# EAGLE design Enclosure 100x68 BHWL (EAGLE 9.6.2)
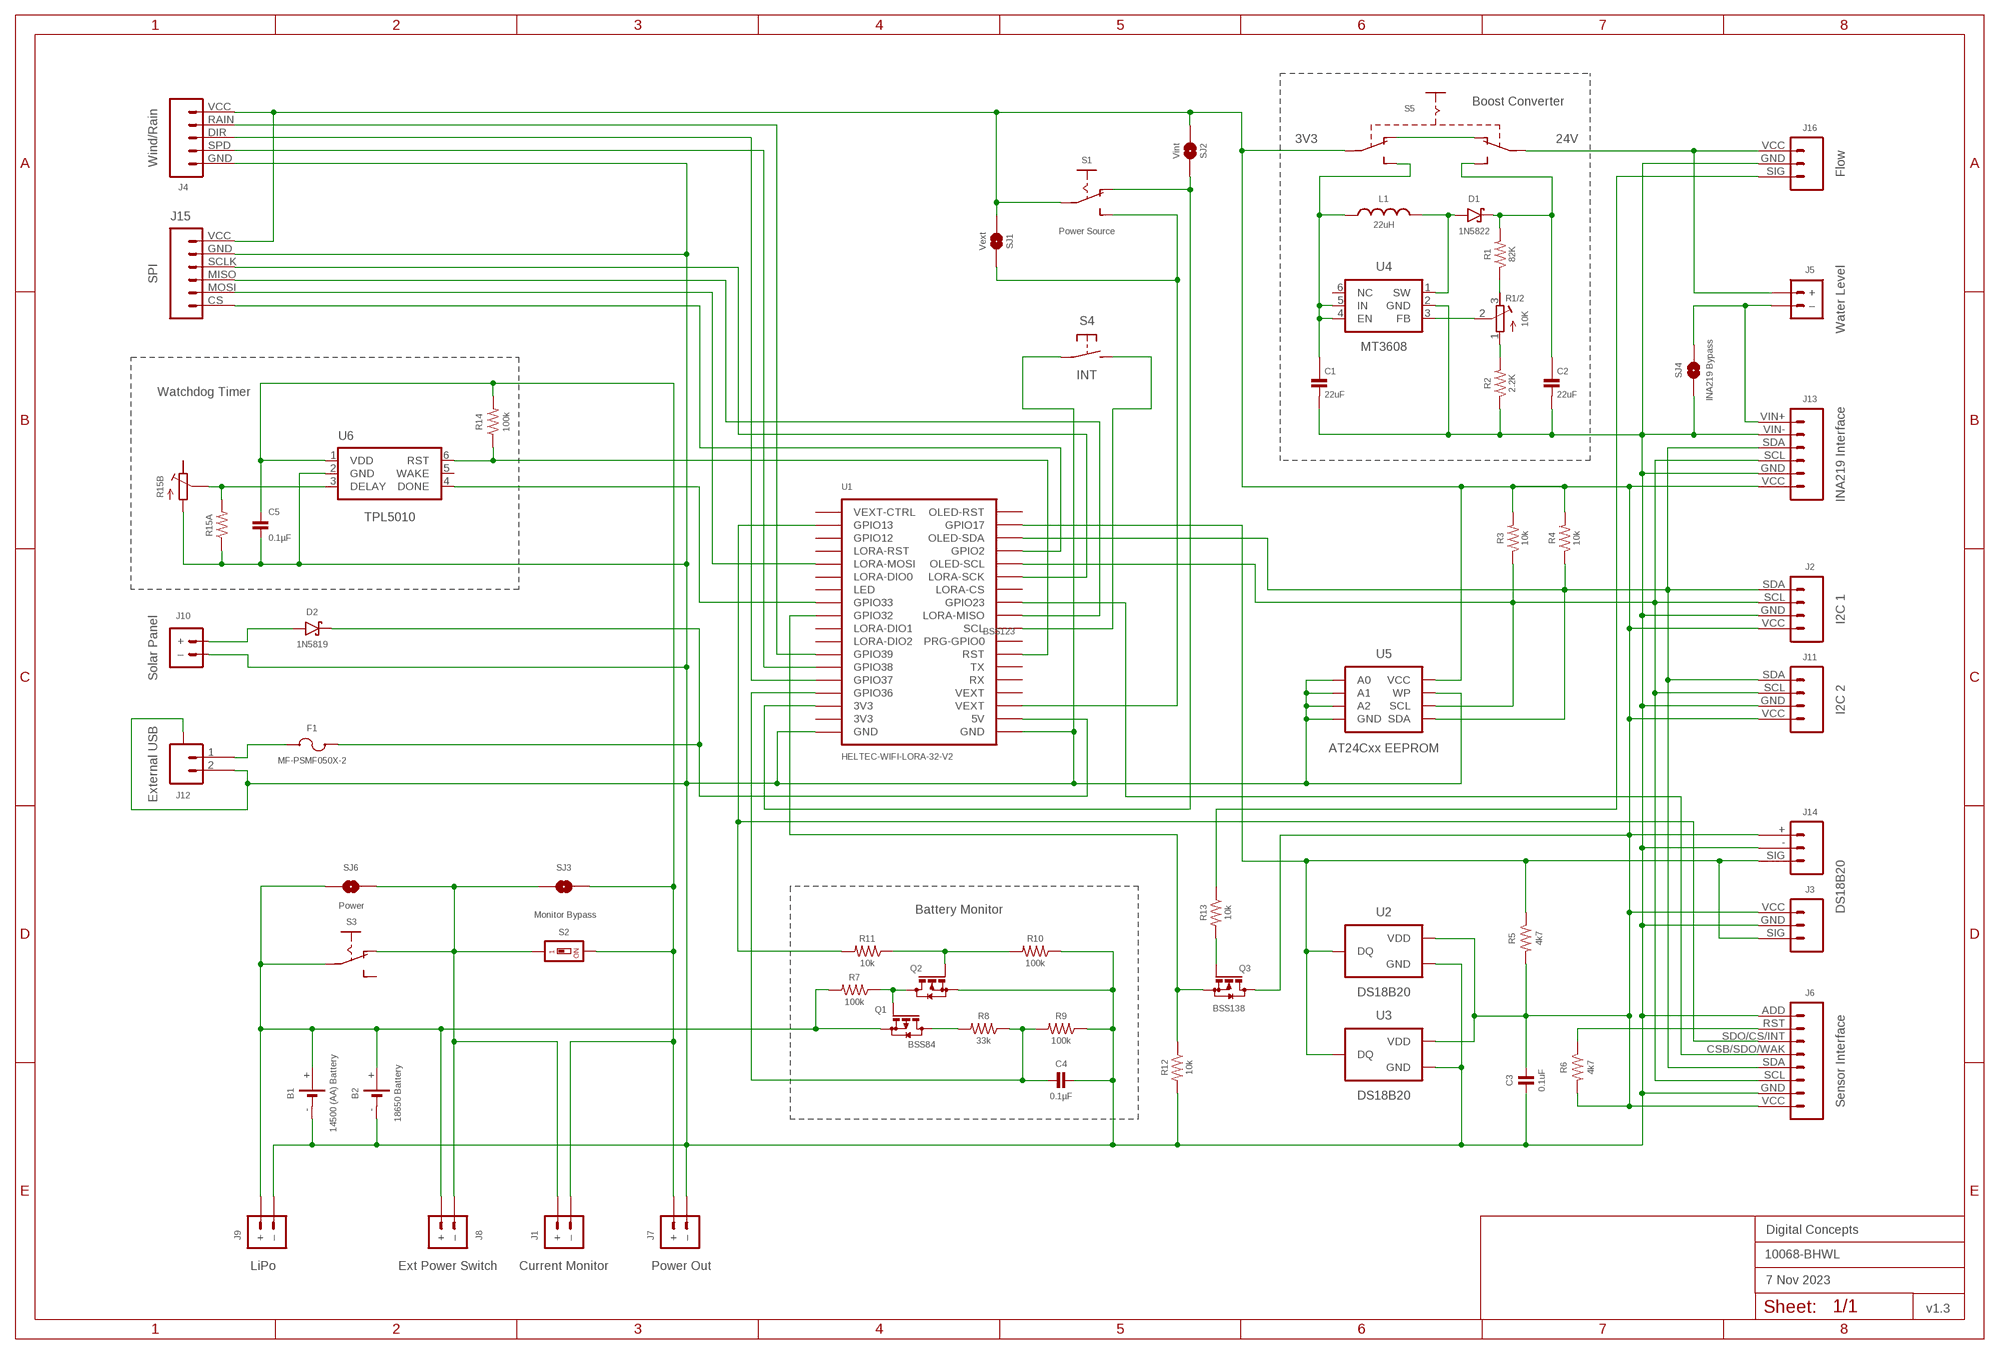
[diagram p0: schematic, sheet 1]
FRAME2 (A3L-LOC): DATE: 7 Nov 2023; OWNER: Digital Concepts; TITLE: 10068-BHWL; VERSION: v1.3

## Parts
B1  14500 (AA) Battery  BATTERY-HOLDER-14500(AA)  [BATTERY-14500]
B2  18650 Battery  BATTERY-HOLDER-18650  [BATTERY-18650]
C1  22uF  CAPACITOR-1206  [C1206]
C2  22uF  CAPACITOR-1206  [C1206]
C3  0.1uF  CAPACITOR-0805  [C0805]
C4  0.1µF  CAPACITOR-0805  [C0805]
C5  0.1µF  CAPACITOR-0805  [C0805]
D1  1N5822  DIODE-SCHOTTKY-1N5822  [DIODE_SMB]
D2  1N5819  1N5819-SOD-123  [SOD-123]
F1  MF-PSMF050X-2  [F0805]
J1  Current Monitor  JST-PH2.0-2-HORIZONTALJST-PTH-2  [JST-PH2.0-2-HORIZONTAL]
J2  I2C 1  JST-PH2.0-4-VERTICAL-I2C  [JST-PH2.0-4-VERTICAL-I2C]
J3  DS18B20  JST-PH2.0-3-VERTICAL-DS18B20  [JST-PH2.0-3-VERTICAL-SIG]
J4  Wind/Rain  JST-PH2.0-5-DUAL-WEATHER  [JST-PH2.0-5-DUAL-WEATHER]
J5  Water Level  JST-PH2.0-2-DUAL-POWERJST-PTH-2  [JST-PH2.0-2-DUAL-POWER]
J6  Sensor Interface  HEADER-1X8-SENSOR  [CONN_08-SENSOR]
J7  Power Out  JST-GH1.25-2-HORIZONTAL-POWER  [JST-GH1.25-2-HORIZONTAL]
J8  Ext Power Switch  JST-PH2.0-2-DUAL-POWERJST-PTH-2  [JST-PH2.0-2-DUAL-POWER]
J9  LiPo  JST-PH2.0-2-HORIZONTAL-POWERJST-PTH-2  [JST-PH2.0-2-HORIZONTAL-POWER]
J10  Solar Panel  JST-PH2.0-2-VERTICAL  [JST-PH2.0-2-VERTICAL=POWER]
J11  I2C 2  JST-PH2.0-I2C-MALE-HORIZONTAL  [JST-PH2.0-4-HORIZONTAL]
J12  External USB  JST-SH1.0-2-SMD-HORIZONTAL  [JST-SH1.0-2-HORIZONTAL]
J13  INA219 Interface  INA219-I2C-MODULE  [CONN_06-INA219]
J14  JST-PH2.0-3-HORIZONTAL-DS18B20  [JST-PH2.0-3-HORIZONTAL-DS18B20]
J15  SPI  JST-PH2.0-6-HORIZONTAL-SPI  [JST-PH2.0-6-HORIZONTAL-SPI]
J16  Flow  JST-XH2.54-3-VERTICAL-SENSOR  [JST-XH2.4-3-VERTICAL-SENSOR]
L1  22uH  INDUCTOR-CDRH104R/6D28L5038P  [CDRH104R+6D28]
Q1  BSS84  [SOT23-3]
Q2  BSS123  MOSFET-BSS123  [SOT23-3]
Q3  BSS138  MOSFET-BSS123  [SOT23-3]
R1  82K  RESISTORR0805  [R0805]
R1/2  10K  RESISTOR-TRIMM-BAOTER-HORIZONTAL  [RTRIM64P]
R2  2.2K  RESISTORR0805  [R0805]
R3  10k  RESISTORR0805  [R0805]
R4  10k  RESISTORR0805  [R0805]
R5  4k7  RESISTORR0805  [R0805]
R6  4k7  RESISTORR0805  [R0805]
R7  100k  RESISTORR0805  [R0805]
R8  33k  RESISTORR0805  [R0805]
R9  100k  RESISTORR0805  [R0805]
R10  100k  RESISTORR0805  [R0805]
R11  10k  RESISTORR0805  [R0805]
R12  10k  RESISTORR0805  [R0805]
R13  10k  RESISTORR0805  [R0805]
R14  100k  RESISTORR0805  [R0805]
R15A  RESISTORR0805  [R0805]
R15B  RESISTOR-TRIMM-33  [RTRIM3*3]
S1  Power Source  SWITCH-SLIDE-SPDT-SMT  [SWITCH-SPDT-SMT]
S2  Monitor Bypass  SWITCH-DIP-SWS001  [SMD-001]
S3  Power  SWITCH-SLIDE-SPDT-PTH  [SWITCH-SPDT-PTH]
S4  INT  SWITCH-MOMENTARY-2-PIN  [SWITCH-2-PAD]
S5  SWITCH-SLIDE-DPDT-PTH-S  [SWITCH-DPDT-PTH]
SJ1  Vext  SJ  [SJ]
SJ2  Vint  SJ-V-2  [SJ-VIA-2]
SJ3  Monitor  SJ  [SJ]
SJ4  INA219 Bypass  SJ  [SJ]
SJ6  Power  SJ  [SJ]
U1  HELTEC-WIFI-LORA-32-V2  [HELTEC-WIFI-LORA-32-V2]
U2  DS18B20  THERMOMETER-DS18B20  [TO-92]
U3  DS18B20  THERMOMETER-DS18B20  [TO-92]
U4  MT3608  [SOT-23-6@1]
U5  AT24Cxx EEPROM  AT24CXX-EEPROM  [SOP-8]
U6  TPL5010  TPL5010DDCR  [SOT-23-6]

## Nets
GND: B1.- B2.- C1.2 C2.2 C3.2 C4.2 C5.2 J2.GND J3.GND J4.GND J6.ADD J6.GND J7.-(–) J9.-(–) J10.-(–) J11.GND J12.2 J12.A@1(A) J12.A@2(A) J13.GND J13.VIN- J14.- J15.GND J16.GND Q2.2(S) R2.1 R9.1 R10.1 R12.2 R15A.1 R15B.1(A) S4.P$1(P) SJ4.1 U1.GND@1(GND) U1.GND@36(GND) U2.1(GND) U3.1(GND) U4.2(GND) U5.P$1(A0) U5.P$2(A1) U5.P$3(A2) U5.P$4(GND) U5.P$7(WP) U6.2(GND)
N$1: D2.A J10.+
N$2: J4.RAIN U1.GPIO39
N$3: J6.CSB/SDO/WAK U1.GPIO23
N$4: J2.SCL J6.SCL J11.SCL J13.SCL R3.1 U1.GPIO15(OLED-SCL) U5.P$6(SCL)
N$5: D2.C F1.1 U1.5V
N$6: D1.A L1.1 U4.1(SW)
N$7: Q1.3(D) R8.2
N$8: C5.1 J1.2(–) J7.+ R14.2 S2.2 SJ3.1 U6.1(VDD)
N$9: J6.RST R6.1
N$10: J4.DIR U1.GPIO37
N$11: J2.SDA J6.SDA J11.SDA J13.SDA R4.1 U1.GPIO4(OLED-SDA) U5.P$5(SDA)
N$12: J4.SPD U1.GPIO38
N$13: S1.3(S) SJ1.1 U1.VEXT@3(VEXT)
N$14: F1.2 J12.1
N$15: J5.-(–) J13.VIN+ SJ4.2
N$16: R1.1 R1/2.3(E)
N$17: S4.P$2(S) U1.GPIO22(SCL)
N$18: C4.1 R8.1 R9.2 U1.GPIO36
N$19: S1.1(O) SJ2.1 U1.3V3@34(3V3)
N$20: J5.+ J16.VCC S5.P$2(P1)
N$21: J1.1(+) J8.-(–) S2.1 S3.1(O) SJ3.2 SJ6.1
N$22: R1/2.2(S) U4.3(FB)
N$23: R1/2.1(A) R2.2
N$24: J3.SIG J14.SIG R5.1 U1.GPIO17 U2.2(DQ) U3.2(DQ)
N$25: C1.1 L1.2 S5.P$6(S2) U4.4(EN) U4.5(IN)
N$26: S5.P$1(O1) S5.P$4(O2)
N$27: J15.SCLK U1.GPIO5(LORA-SCK)
N$28: C2.1 D1.C R1.2 S5.P$3(S1)
N$29: J15.MOSI U1.GPIO27(LORA-MOSI)
N$30: B1.+ B2.+ J8.+ J9.+ Q1.2(S) R7.2 S3.2(P) SJ6.2
N$31: J15.MISO U1.GPIO19(LORA-MISO)
N$32: J6.SDO/CS/INT R11.2 U1.GPIO13
N$33: J15.CS U1.GPIO2
N$34: Q3.1(G) R13.2
N$35: Q1.1(G) Q2.3(D) R7.1
N$36: R15A.2 R15B.2(S) U6.3(DELAY)
N$37: Q2.1(G) R10.2 R11.1
N$38: R14.1 U1.RST U6.6(RST)
N$39: U1.GPIO33 U6.4(DONE)
N$40: Q3.2(S) R12.1 U1.GPIO32
N$42: J16.SIG R13.1
VEXT: C3.1 J2.VCC J3.VCC J4.VCC J6.VCC J11.VCC J13.VCC J14.+ J15.VCC Q3.3(D) R3.2 R4.2 R5.2 R6.2 S1.2(P) S5.P$5(P2) SJ1.2 SJ2.2 SJ2.2@V U2.3(VDD) U3.3(VDD) U5.P$8(VCC)
Unconnected: R15B.3(E) S3.3(S) U1.3V3@35(3V3) U1.GPIO0(PRG-GPIO0) U1.GPIO12 U1.GPIO14(LORA-RST) U1.GPIO16(OLED-RST) U1.GPIO18(LORA-CS) U1.GPIO21(VEXT-CTRL) U1.GPIO25(LED) U1.GPIO26(LORA-DIO0) U1.GPIO34(LORA-DIO2) U1.GPIO35(LORA-DIO1) U1.RX U1.TX U1.VEXT@4(VEXT) U4.6(NC) U6.5(WAKE)

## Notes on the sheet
- Boost Converter
- 3V3 | 24V
- Watchdog Timer
- Battery Monitor

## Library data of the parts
B1 = digitalconcepts:BATTERY-HOLDER-14500(AA): 14500 (AA) battery holder
B2 = digitalconcepts:BATTERY-HOLDER-18650: 18650 Battery Holder
C1 C2 = digitalconcepts:CAPACITOR-1206: 1206 Capacitor
C3-C5 = digitalconcepts:CAPACITOR-0805: 0805 Capacitor
D1 = digitalconcepts:DIODE-SCHOTTKY-1N5822: 1N5822 Schottky Diode SMB
D2 = digitalconcepts:1N5819-SOD-123: 1N5819 Schottky Diode SOD-123
F1 = digitalconcepts:MF-PSMF050X-2: PTC Resettable Fuse
J1 = digitalconcepts:JST-PH2.0-2-HORIZONTAL: PH2.0 2P Right Angle PCB Connector; PROD_ID: CONN-09863; SKU: PRT-09914
J2 = digitalconcepts:JST-PH2.0-4-VERTICAL-I2C: PH2.0 4P I2C Vertical Connector
J3 = digitalconcepts:JST-PH2.0-3-VERTICAL-DS18B20: DS18B20 PH2.0 Vertical PCB Connector
J4 = digitalconcepts:JST-PH2.0-5-DUAL-WEATHER: PH2.0 5P Dual Connector
J5 J8 = digitalconcepts:JST-PH2.0-2-DUAL-POWER: JST PH2.0 2P PTH Dual-Side Connector (Power); PROD_ID: CONN-09863; SKU: PRT-09914
J6 = digitalconcepts:HEADER-1X8-SENSOR: IoT Sensors 1x8 Pin Header for 'Sandwich' IoT Sensors
J7 = digitalconcepts:JST-GH1.25-2-HORIZONTAL-POWER: JST GH1.25 2P PTH Connector (Power)
J9 = digitalconcepts:JST-PH2.0-2-HORIZONTAL-POWER: PH2.0 2P Right Angle PCB Connector; PROD_ID: CONN-09863; SKU: PRT-09914
J10 = digitalconcepts:JST-PH2.0-2-VERTICAL: PH2.0 2P PCB Connector
J11 = digitalconcepts:JST-PH2.0-I2C-MALE-HORIZONTAL: PH2.0 4P (I2C) Right Angle PCB Connector
J12 = digitalconcepts:JST-SH1.0-2-SMD-HORIZONTAL: JST SH1.0 2P SMD Horizontal Connector
J13 = digitalconcepts:INA219-I2C-MODULE: INA219 I2C Module
J14 = digitalconcepts:JST-PH2.0-3-HORIZONTAL-DS18B20: DS18B20 PH2.0 Right Angle PCB Connector
J15 = digitalconcepts:JST-PH2.0-6-HORIZONTAL-SPI: PH2.0 6P Horizontal Connector—SPI
J16 = digitalconcepts:JST-XH2.54-3-VERTICAL-SENSOR: XH2.54 3P Vertical Connector with Sensor Labels
L1 = digitalconcepts:INDUCTOR-CDRH104R/6D28: Inductor; SPICEPREFIX: L
Q1 = digitalconcepts:BSS84: P-CHANNEL MOS FET
Q2 Q3 = digitalconcepts:MOSFET-BSS123: N-CHANNEL MOS FET
R1-R14 R15A = digitalconcepts:RESISTOR: Resistor; SPICEPREFIX: R
R1/2 = digitalconcepts:RESISTOR-TRIMM-BAOTER-HORIZONTAL: Trimm Resistor - Horizontal BAOTER
R15B = digitalconcepts:RESISTOR-TRIMM-3*3: Trimm Resistor - 3*3 SMD
S1 = digitalconcepts:SWITCH-SLIDE-SPDT-SMT: Mini Sliding Switch SPDT SMT
S2 = digitalconcepts:SWITCH-DIP-SWS001: SMD Dip Switch 1 pol.
S3 = digitalconcepts:SWITCH-SLIDE-SPDT-PTH: Mini Sliding Switch SPDT PTH
S4 = digitalconcepts:SWITCH-MOMENTARY-2-PIN: 2 Pin Momentary Switch
S5 = digitalconcepts:SWITCH-SLIDE-DPDT-PTH-S: Switch DPDT PTH-S
SJ1 SJ3 SJ4 SJ6 = digitalconcepts:SJ: Solder Jumper
SJ2 = digitalconcepts:SJ-V-2: Solder Jumper with Pad Vias
U1 = digitalconcepts:HELTEC-WIFI-LORA-32-V2: Heltec WiFi LoRa 32 Development Board V2
U2 U3 = digitalconcepts:THERMOMETER-DS18B20: Digital Thermometer -55C-125C TO92-3; AVAILABILITY: Bad; DESCRIPTION: Temperature Sensor Digital, Local -55°C ~ 125°C 12 b 8-uMAX; MF: Maxim Integrated; MP: DS18B20; PACKAGE: TO-92 Maxim Integrated; PRICE: None
U4 = digitalconcepts:MT3608: MT3608 DC-DC Step-Up Voltage Converter
U5 = digitalconcepts:AT24CXX-EEPROM: AT24Cxx EEPROM SOP-8
U6 = digitalconcepts:TPL5010DDCR: TPL5010 Nano-Power System Timer with Watchdog

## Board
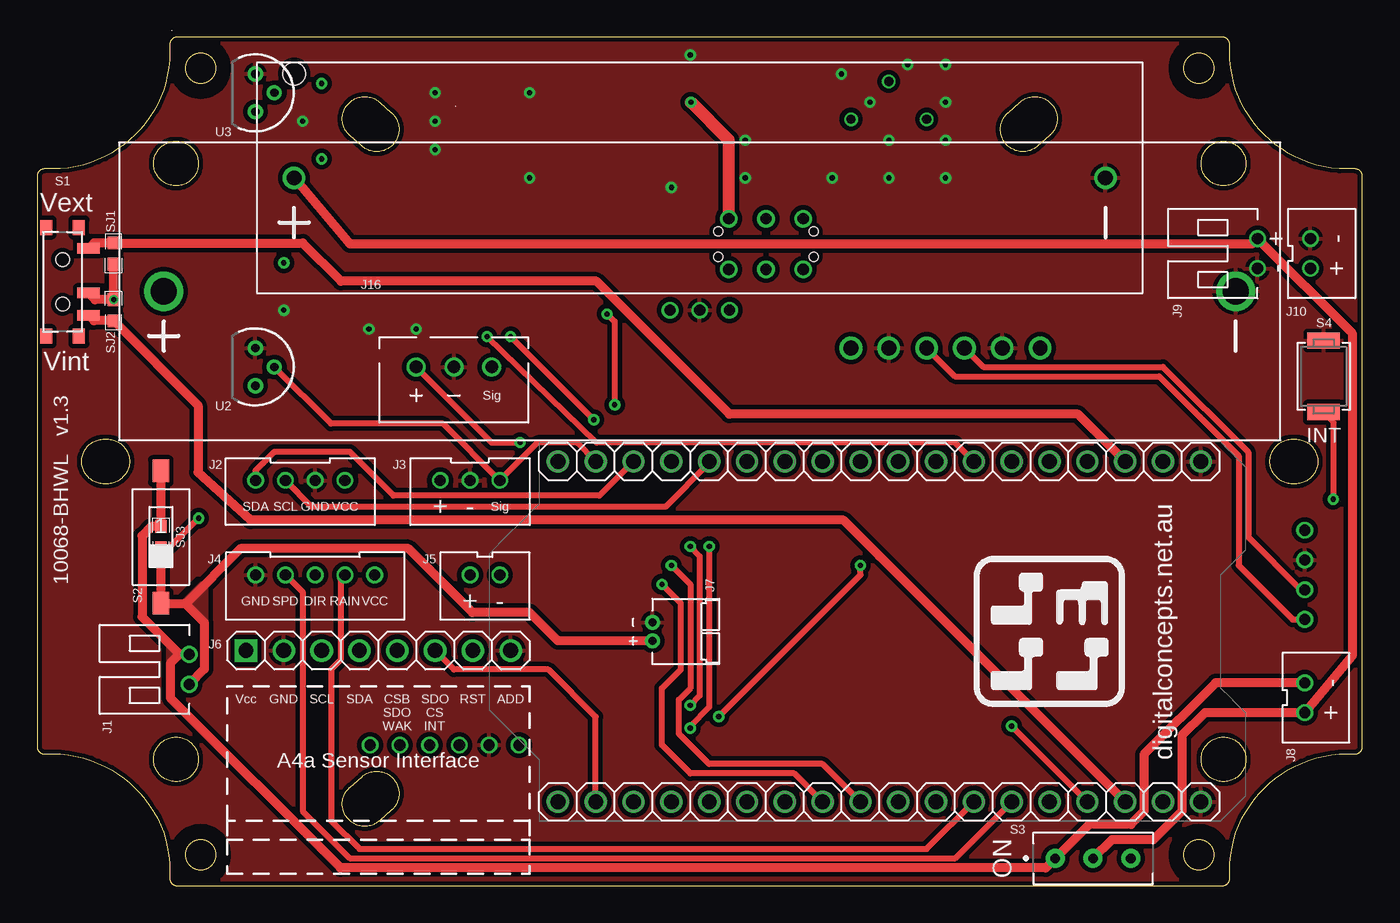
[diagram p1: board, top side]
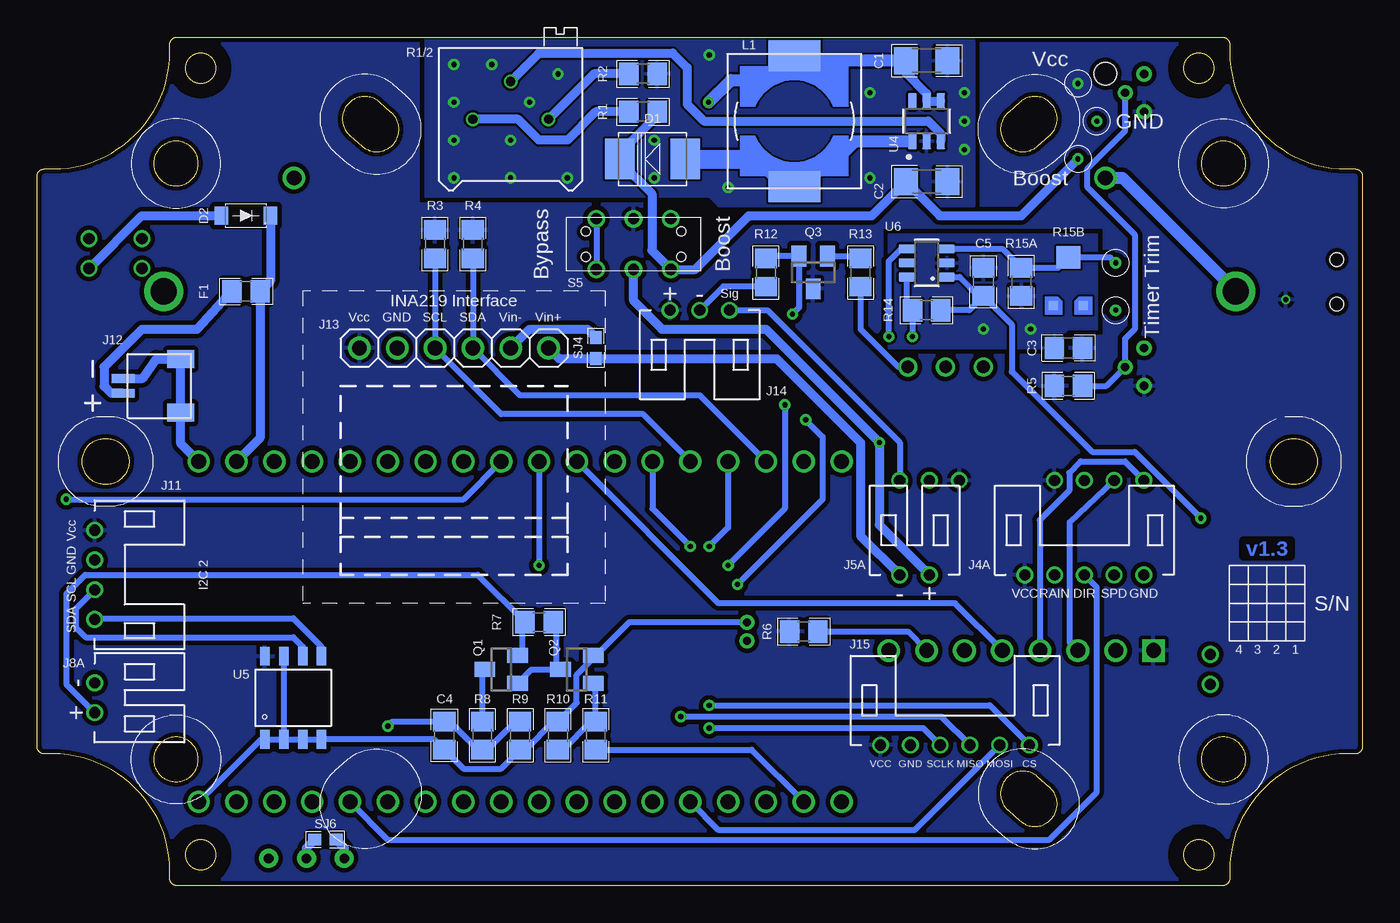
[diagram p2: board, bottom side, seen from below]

Size 89 x 57 mm. Coordinates in mm from the lower left corner, seen from the top.
Outline: 1134 segments
Outline: circle at 10.97,2.08 radius 1.02
Outline: circle at 10.97,54.92 radius 1.02
Outline: circle at 78.03,54.92 radius 1.02
Outline: circle at 78.03,2.08 radius 1.02
Copper layers (1*16): Top 0.035mm / dielectric 1.5mm / Bottom 0.035mm
Design rules "default *": minimum track width 6mil, minimum drill 0.35mm, track to track 6mil, track to pad 6mil, pad to pad 6mil, via to via 6mil, smd to smd 6mil, copper to edge 6mil, drill to drill 6mil, minimum pad ring 1mil, minimum via ring 8mil, stop-mask expansion 4mil, vias tented up to drill 0mil, thermal gap 10mil

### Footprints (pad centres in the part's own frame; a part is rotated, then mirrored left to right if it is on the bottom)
BATTERY-14500 = drill 1: + -27.25,0; - 27.25,0 | hole 1.524: -27.25,7
BATTERY-18650 = drill 1.75: + -36,0; - 36,0
C1206 = smd 1.6 x 1.8: 1 -1.4,0; 2 1.4,0
C0805 = smd 1.3 x 1.5: 1 -0.95,0; 2 0.95,0
DIODE_SMB = smd 2 x 2.7: A 2.2,0; C -2.2,0
SOD-123 = smd 0.91 x 1.22: A -1.65,0; C 1.65,0
F0805 = smd 1.3 x 1.5: 1 -0.95,0; 2 0.95,0
JST-PH2.0-2-HORIZONTAL = drill 0.75: 1 1,0; 2 -1,0
JST-PH2.0-4-VERTICAL-I2C = drill 0.75: GND 1,0; SCL -1,0; SDA -3,0; VCC 3,0
JST-PH2.0-3-VERTICAL-SIG = drill 0.75: GND 0,0; SIG 2,0; VCC -2,0
JST-PH2.0-5-DUAL-WEATHER = drill 0.75: DIR 0,0; GND 4,0; RAIN -2,0; SPD 2,0; VCC -4,0
JST-PH2.0-2-DUAL-POWER = drill 0.75: + 1,0; - -1,0
CONN_08-SENSOR = drill 1 pad 1.524: ADD 17.78,0; CSB/SDO/WAK 10.16,0; GND 2.54,0; RST 15.24,0; SCL 5.08,0; SDA 7.62,0; SDO/CS/INT 12.7,0 | drill 1 pad 1.524 square: VCC 0,0
JST-GH1.25-2-HORIZONTAL = drill 0.55 pad 1.016: + -0.625,0; - 0.625,0
JST-PH2.0-2-HORIZONTAL-POWER = drill 0.75: + 1,0; - -1,0
JST-PH2.0-2-VERTICAL=POWER = drill 0.75: + -1,0; - 1,0
JST-PH2.0-4-HORIZONTAL = drill 0.75: GND -1,0; SCL 1,0; SDA 3,0; VCC -3,0
JST-SH1.0-2-HORIZONTAL = smd 0.6 x 1.55: 1 -0.5,2.54; 2 0.5,2.54 | smd 1.2 x 1.8: A@1 -1.8,-1.335; A@2 1.8,-1.335
CONN_06-INA219 = drill 1 pad 1.524: GND 2.54,0; SCL 5.08,0; SDA 7.62,0; VCC 0,0; VIN+ 12.7,0; VIN- 10.16,0
JST-PH2.0-3-HORIZONTAL-DS18B20 = drill 0.75: + 2,0; - 0,0; SIG -2,0
JST-PH2.0-6-HORIZONTAL-SPI = drill 0.75: CS 5,0; GND -3,0; MISO 1,0; MOSI 3,0; SCLK -1,0; VCC -5,0
JST-XH2.4-3-VERTICAL-SENSOR = drill 0.85: GND 0,0; SIG 2.54,0; VCC -2.54,0
CDRH104R+6D28 = smd 2.1 x 3.5: 1 -4.4,0; 2 4.4,0
SOT23-3 = smd 1 x 1.4: 1 -0.95,-1.1; 2 0.95,-1.1; 3 0,1.1
R0805 = smd 1.3 x 1.5: 1 -0.95,0; 2 0.95,0
RTRIM64P = drill 0.61: 1 0,-2.54; 2 2.54,0; 3 0,2.54
RTRIM3*3 = smd 0.6 x 0.6: 1 -1,-1.6; 3 1,-1.6 | smd 1.6 x 1.5: 2 0,1.65
SWITCH-SPDT-SMT = smd 0.7 x 1.5: 1 2.25,1.75; 2 0.75,1.75; 3 -2.25,1.75 | smd 1 x 0.8: GND@1 3.65,-1.1; GND@2 3.65,1.1; GND@3 -3.65,1.1; GND@4 -3.65,-1.1 | hole 0.9: -1.5,0; 1.5,0
SMD-001 = smd 1.1 x 1.5: 1 0,-4.45; 2 0,4.45
SWITCH-SPDT-PTH = drill 0.65 pad 1.27: 1 -2.54,0; 2 0,0; 3 2.54,0
SWITCH-2-PAD = smd 1.067 x 2.184: P$1 -2.4,0; P$2 2.4,0
SWITCH-DPDT-PTH = drill 0.75 pad 1.19: P$1 -1.7,2.5; P$2 -1.7,0; P$3 -1.7,-2.5; P$4 1.7,2.5; P$5 1.7,0; P$6 1.7,-2.5 | hole 0.6: 0.85,3.2; -0.85,3.2; 0.85,-3.2; -0.85,-3.2
SJ = smd 0.864 x 0.762: 1 -0.711,0; 2 0.711,0
SJ-VIA-2 = smd 0.864 x 0.762: 1 -0.711,0; 2 0.711,0 | drill 0.35 pad 0.61: 2@V 0.711,0
HELTEC-WIFI-LORA-32-V2 = drill 1: 3V3@34 -22.86,5.08; 3V3@35 -22.86,2.54; 5V 0,2.54; GND@1 0,0; GND@36 -22.86,0; GPIO0 0,17.78; GPIO2 0,35.56; GPIO4 0,38.1; GPIO5 0,30.48; GPIO12 -22.86,38.1; GPIO13 -22.86,40.64; GPIO14 -22.86,35.56; GPIO15 0,33.02; GPIO16 0,43.18; GPIO17 0,40.64; GPIO18 0,27.94; GPIO19 0,22.86; GPIO21 -22.86,43.18; GPIO22 0,20.32; GPIO23 0,25.4; GPIO25 -22.86,27.94; GPIO26 -22.86,30.48; GPIO27 -22.86,33.02; GPIO32 -22.86,22.86; GPIO33 -22.86,25.4; GPIO34 -22.86,17.78; GPIO35 -22.86,20.32; GPIO36 -22.86,7.62; GPIO37 -22.86,10.16; GPIO38 -22.86,12.7; GPIO39 -22.86,15.24; RST 0,15.24; RX 0,10.16; TX 0,12.7; VEXT@3 0,5.08; VEXT@4 0,7.62
TO-92 = drill 0.55 pad 1.016: 1 -1.27,0; 2 0,1.27; 3 1.27,0
SOT-23-6@1 = smd 1.1 x 0.6: 1 -1.35,0.95; 2 -1.35,0; 3 -1.35,-0.95; 4 1.35,-0.95; 5 1.35,0; 6 1.35,0.95
SOP-8 = smd 0.635 x 1.27: P$1 -1.905,-2.794; P$2 -0.635,-2.794; P$3 0.635,-2.794; P$4 1.905,-2.794; P$5 1.905,2.794; P$6 0.635,2.794; P$7 -0.635,2.794; P$8 -1.905,2.794
SOT-23-6 = smd 1.1 x 0.6: 1 -1.35,0.95; 2 -1.35,0; 3 -1.35,-0.95; 4 1.35,-0.95; 5 1.35,0; 6 1.35,0.95

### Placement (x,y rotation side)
B1  44.5,47.55 0 top
B2  44.5,39.93 0 top
C1  29.26,55.42 0 bottom
C2  29.26,47.3 0 bottom
C3  19.73,36.12 180 bottom
C4  61.64,10.08 270 bottom
C5  25.45,40.56 90 bottom
D1  47.67,48.82 0 bottom
D2  74.98,45.01 0 bottom
F1  74.98,39.93 180 bottom
J1  10.21,14.53 90 top
J2  17.67,27.23 0 top
J3  29.07,27.23 0 top
J4  18.67,20.88 0 bottom
J5  30.07,20.88 0 bottom
J6  14.02,15.8 0 top
J7  41.32,17.07 90 top
J8  85.14,12.62 270 bottom
J9  81.96,42.47 90 top
J10  85.52,42.47 90 top
J11  85.14,20.88 270 bottom
J12  80.69,33.58 90 bottom
J13  67.36,36.12 0 bottom
J14  44.5,38.66 180 bottom
J15  27.35,9.45 0 bottom
J16  27.99,34.85 0 top
L1  38.15,51.36 90 bottom
Q1  57.83,14.53 90 bottom
Q2  52.75,14.53 90 bottom
Q3  36.88,41.2 180 bottom
R1  48.31,51.99 0 bottom
R1/2  57.2,51.49 90 bottom
R2  48.31,54.53 180 bottom
R3  62.28,43.1 90 bottom
R4  59.74,43.1 90 bottom
R5  19.73,33.58 180 bottom
R6  37.51,17.07 180 bottom
R7  55.29,17.7 180 bottom
R8  59.1,10.08 90 bottom
R9  56.56,10.08 90 bottom
R10  54.02,10.08 270 bottom
R11  51.48,10.08 270 bottom
R12  40.05,41.2 270 bottom
R13  33.7,41.2 90 bottom
R14  29.26,38.66 0 bottom
R15A  22.91,40.56 90 bottom
R15B  19.73,40.56 0 bottom
S1  1.7,40.56 270 top
S2  8.3,23.42 180 top
S3  70.92,1.83 0 top
S4  86.41,34.21 270 top
S5  48.94,43.1 90 bottom
SJ1  5.13,42.47 270 top
SJ2  5.13,38.66 90 top
SJ3  8.3,23.42 90 top
SJ4  51.48,36.12 270 bottom
SJ6  69.65,3.1 180 bottom
U1  78.15,28.5 90 top
U2  14.65,34.85 270 top
U3  14.65,53.26 270 top
U4  29.26,51.36 90 bottom
U5  71.8,12.62 0 bottom
U6  29.26,41.83 180 bottom

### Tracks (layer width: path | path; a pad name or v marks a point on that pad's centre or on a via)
$X
  cutout Bottom: 10.97,56.95 arc180 10.97,52.88 arc180
$X1
  cutout Bottom: 78.03,56.95 arc180 78.03,52.88 arc180
$X2
  cutout Top: 78.03,4.12 arc180 78.03,0.05 arc180
$X3
  cutout Top: 10.97,4.12 arc180 10.97,0.05 arc180
$X4
  cutout Top: 10.97,56.95 arc180 10.97,52.88 arc180
$X5
  cutout Top: 78.03,56.95 arc180 78.03,52.88 arc180
$X6
  cutout Bottom: 78.03,4.12 arc180 78.03,0.05 arc180
$X7
  cutout Bottom: 10.97,4.12 arc180 10.97,0.05 arc180
GND  (via drill 0.35)
  Bottom 0.406: U5.P$7 U5.P$2 | U5.P$2 U5.P$1 73.96,9.83 U1.GND@36 | U5.P$2 U5.P$3 U5.P$4 62.34,9.83 C4.2 60.37,7.86 57.83,7.86 R9.1 56.21,9.13 54.31,11.03 R10.1 52.76,12.3 52.76,14.18 51.65,15.28 | 51.65,15.28 Q2.2 | J7.- 49.24,17.69 51.65,15.28 | R12.2 42.91,40.25 J14.-
  Bottom 0.61: J12.2 81.93,34.08 81,35.38 J12.A@2 J12.A@1 79.36,29.7 U1.GND@1 | J13.VIN- 55.93,37.39 52.04,37.39 SJ4.1
  other vias: 26.72,53.26 54.02,54.53 61.01,52.63 47.55,50.09 47.55,47.55 53.39,47.55 57.2,47.55 57.2,50.09 61.01,47.55 61.01,50.09 58.47,55.17 26.72,51.36 55.93,52.63 61.01,55.17 43.86,55.8 33.07,53.26 33.07,47.55 26.72,49.45 17.83,51.36 42.59,46.91 22.27,37.39 25.45,37.39 16.56,38.66
  pour Top (isolate 0.305, rank 2): -1.65,58.87 -1.65,-1.92 90.59,-1.92 90.59,58.87
  pour Bottom: 26.08,57.07 26.08,45.64 43.23,45.64 43.86,46.28 62.91,46.28 62.91,57.07
  pour Bottom: 17.83,37.39 19.73,37.39 21,36.12 31.8,36.12 31.8,43.74 17.83,43.74
N$1
  Bottom 0.61: J10.+ 81.98,45.01 D2.A
N$2
  Top 0.406: J4.RAIN 20.37,20.58 20.37,15.16 19.73,14.53 19.73,4.37 21.64,2.46 59.74,2.46 U1.GPIO39
N$3
  Bottom 0.406: J6.CSB/SDO/WAK 27.35,18.97 43.23,18.97 U1.GPIO23
N$4
  Top 0.406: J13.SCL 63.55,34.85 75.61,34.85 81.33,29.13 81.33,23.42 84.87,19.88 J11.SCL | U1.GPIO15 45.13,28.39 42.19,25.45 18.45,25.45 J2.SCL
  Bottom 0.406: J2.SCL 19.66,24.41 19.66,16.36 J6.SCL | U5.P$6 71.17,16.05 71.8,16.69 85.76,16.69 86.41,17.34 86.41,18.61 J11.SCL | R3.1 J13.SCL 57.83,31.67 48.31,31.67 U1.GPIO15
N$5
  Bottom 0.61: D2.C 73.33,40.63 F1.1 74.03,30.08 U1.5V
N$6
  Bottom 0.152: U4.1 30.4,50.01
  Bottom 0.813: 40.68,48.82 38.96,47.11 L1.1 36.84,48.27 35.79,48.27 34.05,50.01 30.4,50.01
  Bottom 1.27: D1.A 40.68,48.82
N$7
  Bottom 0.406: Q1.3 59.1,14.36 R8.2
N$8  (via drill 0.35)
  Top 0.406: v10.84,24.69 8.86,22.71 SJ3.1
  Top 0.61: J1.2 11.23,14.55 11.23,17.67 9.96,18.94 | 9.96,18.94 9.93,18.97 S2.2 SJ3.1 | 9.96,18.94 13.66,22.65 24.94,22.65 29.24,18.35 33.07,18.35 34.97,16.44 J7.+
  Bottom 0.406: U6.1 27.04,40.88 25.77,39.61 C5.1 | C5.1 26.4,38.66 R14.2 | C5.1 23.54,37.71 23.54,34.54 18.14,29.13 15.28,29.13 10.84,24.7 v10.84,24.69
  pour Top (no thermals): 9.93,18.98 11.23,17.7 11.23,20.26
N$9
  Bottom 0.406: J6.RST 30.53,17.07 R6.1
N$10
  Bottom 0.406: U1.GPIO37 65.45,3.1 21,3.1 17.83,6.27 17.83,20.04 J4.DIR
N$11
  Top 0.406: J13.SDA 61.64,34.21 75.36,34.21 80.69,28.88 80.69,21.51 84.33,17.88 J11.SDA | U1.GPIO4 37.77,26.21 23.93,26.21 21,29.13 15.92,29.13 14.67,27.88 J2.SDA
  Bottom 0.406: J6.SDA 21.66,15.82 21.66,24.56 19.68,26.54 19.68,27.73 18.92,28.5 15.94,28.5 J2.SDA | J11.SDA 85.06,17.96 71.8,17.96 69.9,16.05 U5.P$5 | R4.1 J13.SDA 56.56,32.94 44.5,32.94 U1.GPIO4
N$12
  Top 0.406: J4.SPD 17.83,19.72 17.83,5 20.98,1.85 61.67,1.85 U1.GPIO38
N$13
  Top 0.61: S1.3 3.82,43.18 SJ1.1 17.83,43.18 20.41,40.6 37.55,40.6 46.48,31.67 69.9,31.67 U1.VEXT@3
N$14
  Bottom 0.61: J12.1 84.02,33.08 84.5,33.56 84.5,34.85 81.96,37.39 78.26,37.39 F1.2
N$15
  Bottom 0.61: J5.- 33.69,23.5 33.7,29.77 39.34,35.41 SJ4.2 53.95,35.41 J13.VIN+
N$16
  Bottom 0.61: R1.1 51.48,51.99 53.39,50.09 55.29,50.09 56.69,51.49 R1/2.3
N$17  (via drill 0.35)
  Top 0.406: S4.P$2 87.04,31.18 v87.04,25.96
  Bottom 0.406: v87.04,25.96 60.37,25.96 U1.GPIO22
N$18  (via drill 0.35)
  Top 0.406: U1.GPIO36 v65.45,10.72
  Bottom 0.406: R9.2 56.87,11.03 58.77,9.13 R8.1 59.38,9.13 61.29,11.03 C4.1 65.14,11.03 v65.45,10.72
N$19
  Top 0.61: S1.1 3.82,37.95 SJ2.1 10.81,32.27 10.81,27.77 14.34,24.56 54.15,24.56 56.56,22.15 U1.3V3@34
N$20  (via drill 0.35)
  Top 0.406: J16.VCC 30.53,29.77 v32.43,29.77
  Bottom 0.61: S5.P$2 48.94,39.29 47.04,37.39 40.05,37.39 v32.43,29.77 32.43,24.24 J5.+
N$21
  Top 0.61: S2.1 SJ3.2 7.67,24.13 7.03,23.5 7.03,18.07 9.57,15.53 J1.1 9.55,15.53 8.94,14.92 8.94,12.62 20.37,1.19 67.74,1.19 S3.1 70.66,4.12 73.46,4.12 74.34,5 74.34,8.81 79.15,13.62 J8.-
  Bottom 0.61: SJ6.1 68.38,2.54 S3.1
  pour Top (no thermals): 9.55,15.55 8.94,16.16 8.94,14.94
N$22
  Bottom 0.61: U4.3 28.31,50.51 29.16,51.36 44.21,51.36 45.35,52.5 45.35,54.95 46.33,55.93 55.29,55.93 R1/2.2
N$23
  Bottom 0.61: R1/2.1 51.61,54.53 R2.2
N$24
  Top 0.406: U2.2 19.73,31.04 27.26,31.04 J3.SIG 33.61,29.77 36.24,29.77 U1.GPIO17
  Bottom 0.406: J3.SIG 31.07,29.77 39.96,38.66 J14.SIG | R5.1 17.19,33.58 U2.2 15.92,36.75 15.29,37.39 15.29,43.74 18.46,46.91 18.46,48.18 15.92,50.72 U3.2
N$25  (via drill 0.35)
  Top 0.813: v43.9,52.63 46.44,50.09 S5.P$6
  Bottom 0.61: C1.1 30.66,54.61 29.26,53.21 U4.5 U4.4
  Bottom 0.813: C1.1 38.04,55.42 L1.2 38.99,55.36 39.98,54.12 42.41,54.12 v43.9,52.63
N$26
  Bottom 0.406: S5.P$4 S5.P$1
N$27  (via drill 0.35)
  Top 0.406: v45.13,22.78 45.13,11.99 43.86,10.72 v43.86,10.59
  Bottom 0.406: U1.GPIO5 47.67,25.32 v45.13,22.78 | v43.86,10.59 29.5,10.59 J15.SCLK
N$28  (via drill 0.35)
  Bottom 0.61: v19.1,48.82 22.91,45.01 28.37,45.01 C2.1 32.95,45.01 41.2,45.01 44.81,41.4 S5.P$3 47.71,42.67 47.71,46.48 49.87,48.64 D1.C 49.87,49.23 47.36,51.74 R1.2
N$29
  Bottom 0.406: J15.MOSI 30.07,3.73 43.23,3.73 U1.GPIO27
N$30
  Top 0.61: B1.+ 21,43.1 81.6,43.1 J9.+ 88.31,37.12 88.31,15.43 J8.+ 78.42,11.62 76.88,10.08 76.88,5 74.98,3.1 72.19,3.1 S3.2
  Bottom 0.406: Q1.2 56.44,15.78 56.44,17.51 R7.2 59.42,20.88 85.77,20.88 87.04,19.61 87.04,13.53 J8.+
  Bottom 0.61: SJ6.2 70.92,2.54 S3.2
  Bottom 0.813: B1.+ 16.12,47.55 B2.+
N$31  (via drill 0.35)
  Top 0.406: v45.77,11.35 55.29,20.88 v55.29,21.51
  Bottom 0.406: U1.GPIO19 v55.29,21.51 | J15.MISO 28.26,11.35 v45.77,11.35
N$32
  Top 0.406: U1.GPIO13 37.51,11.35 34.34,14.53 27.99,14.53 J6.SDO/CS/INT
  Bottom 0.406: U1.GPIO13 41.01,9.13 R11.2
N$33  (via drill 0.35)
  Top 0.406: v43.86,22.78 44.5,22.15 44.5,12.75 v43.86,12.12
  Bottom 0.406: v43.86,22.78 42.59,24.05 U1.GPIO2 | J15.CS 25.02,12.12 v43.86,12.12
N$34
  Bottom 0.406: Q3.1 33.85,42.3 R13.2
N$35
  Bottom 0.406: Q1.1 55.78,14.53 Q2.3 54.15,14.83 54.15,17.51 R7.1
N$36  (via drill 0.35)
  Bottom 0.406: U6.3 24.18,42.78 R15A.2 20.43,41.51 R15B.2 16.94,42.21 v16.56,41.83
N$37
  Bottom 0.406: R10.2 53.69,9.13 51.79,11.03 R11.1 51.48,13.41 Q2.1
N$38  (via drill 0.35)
  Top 0.406: U1.RST 61.64,29.77 37.58,29.77 v30.21,36.88
  Bottom 0.406: U6.6 30.61,39.06 R14.1 v30.21,36.88
N$39  (via drill 0.35)
  Top 0.406: U1.GPIO33 50.85,7.54 43.86,7.54 41.96,9.45 41.96,13.26 43.23,14.53 43.23,18.97 v41.96,20.24 | v37.39,31.29 v31.8,36.88
  Bottom 0.406: v37.39,31.29 36.24,30.15 36.24,25.96 v41.96,20.24 | U6.4 30.97,42.78 31.8,41.95 v31.8,36.88
N$40  (via drill 0.35)
  Top 0.406: v38.28,38.41 38.78,37.9 v38.78,32.31 | v42.59,21.51 43.86,20.24 43.86,13.26 43.1,12.5 43.1,10.21 45.13,8.18 52.75,8.18 U1.GPIO32
  Bottom 0.406: v38.78,32.31 38.78,25.32 v42.59,21.51 | v38.28,38.41 37.83,38.85 Q3.2 39.9,42.3 R12.1
N$42
  Bottom 0.406: R13.1 33.7,37.39 31.16,34.85 J16.SIG
VEXT  (via drill 0.35)
  Top 0.61: S1.2 3.89,39.37 SJ2.2@V SJ1.2
  other vias: 19.1,53.9
  pour Bottom (isolate 0.305, rank 2): -0.65,57.87 -0.65,-0.92 89.59,-0.92 89.59,57.87

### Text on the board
Bottom: v1.3
tPlace: 10068-BHWL v1.3 | digitalconcepts.net.au | Vcc | GND | SCL | SDA | RST | ADD | CSB / SDO / WAK | SDO / CS / INT
bPlace: Vin+ | Vin- | SDA | SCL | GND | Vcc | S/N | 1 | 2 | 3 | 4
tNames: Vext | Vint | A4a Sensor Interface | ON
bNames: Vcc | GND | Boost | Boost | Bypass | Timer Trim | Vcc | GND | J4A | J5A | SCL | SDA | J8A
bValues: Wind/Rain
